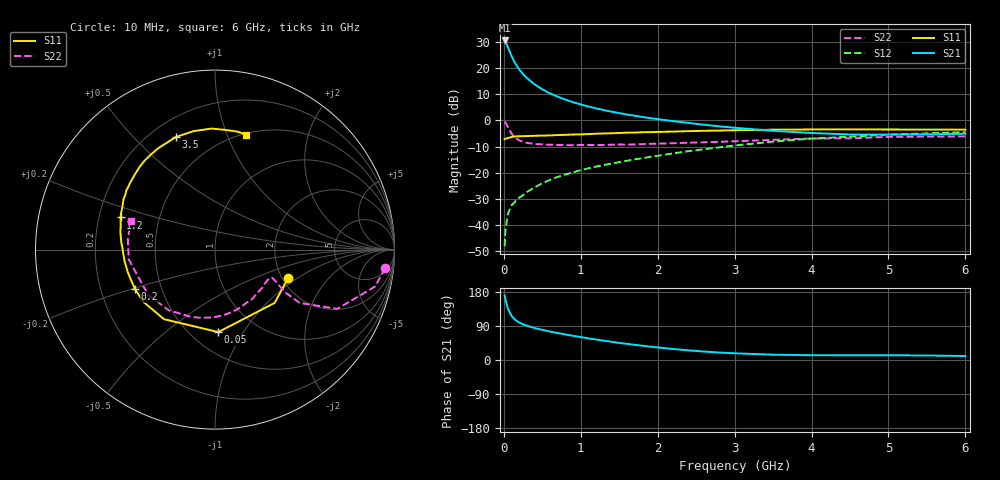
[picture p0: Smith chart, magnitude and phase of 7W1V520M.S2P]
! Infineon Technologies  Discrete & RF Semiconductors
! BFS17W
! Si NPN RF Bipolar Junction Transistor in SOT323
! VCE = 1.5 V  IC = 20 mA
! Common Emitter S-Parameters:  August  1999
# GHz  S  MA  R  50
!  f  S11  S21  S12  S22
! GHz  MAG  ANG  MAG  ANG  MAG  ANG  MAG  ANG
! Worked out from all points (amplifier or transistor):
!   36 points, 10 MHz to 6 GHz, reference 50 ohm
!   highest |S21| = 30.6 dB at 10 MHz (marker M1)
!   |S21| within 3 dB of that: start of sweep to 58.85 MHz
!   unconditionally stable (mu >= 1): 219.1 MHz to end of sweep
!   at 250 MHz: K = 1.08, MAG = 21.5 dB, |S12| = -28.6 dB
!   at 1.4 GHz: K = 1.28, MAG = 6.7 dB, |S12| = -16.5 dB
!   at 6 GHz: K = 1.11, MAG = -2.3 dB, |S12| = -4.5 dB
!   S11 on the Smith chart (normalised r, x): 10 MHz: 2.14, -0.85; 50 MHz: 0.67, -0.78; 200 MHz: 0.35, -0.20; 1.2 GHz: 0.29, +0.15; 3.5 GHz: 0.30, +0.67; 6 GHz: 0.51, +1.18
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0.01  0.4366 -21.6  34.02 170.0  0.0039 83.4  0.9538 -6.2
0.02  0.4456 -41.8  32.74 159.9  0.0075 74.6  0.9152 -13.0
0.05  0.4599 -87.7  25.94 136.8  0.0159 61.6  0.7565 -25.9
0.1  0.4806 -126.2  17.05 116.3  0.0235 54.6  0.5571 -32.2
0.15  0.4944 -144.1  12.26 105.5  0.0282 55.6  0.4611 -31.4
0.2  0.4971 -153.9  9.496 99.0  0.0332 58.4  0.4148 -29.5
0.25  0.498 -160.8  7.702 94.2  0.0371 60.0  0.3861 -27.9
0.3  0.5018 -165.5  6.476 90.5  0.0425 61.5  0.3724 -27.1
0.4  0.5078 -172.6  4.908 84.3  0.0523 63.7  0.3533 -26.3
0.5  0.5118 -177.6  3.947 79.5  0.0624 66.1  0.3469 -26.7
0.6  0.5159 178.9  3.293 75.1  0.0727 67.0  0.342 -27.9
0.7  0.524 175.4  2.845 71.1  0.0827 67.7  0.3388 -30.0
0.9  0.5368 169.3  2.232 63.8  0.1013 68.1  0.3358 -34.9
1.1  0.5481 163.6  1.846 57.0  0.1211 68.0  0.3377 -41.0
1.2  0.5561 161.2  1.701 54.0  0.1305 67.7  0.3373 -44.3
1.6  0.5828 150.8  1.297 42.6  0.1689 67.4  0.3439 -58.2
2.2  0.6115 137.1  0.97 29.0  0.2334 65.6  0.3662 -80.5
2.8  0.6396 123.7  0.77 19.7  0.3049 61.2  0.3889 -102.8
3.5  0.6643 109.1  0.632 14.0  0.3931 53.7  0.4251 -127.4
4.5  0.6747 91.7  0.538 12.4  0.4891 40.4  0.4543 -161.0
5.5  0.669 79.4  0.54 11.9  0.5658 28.6  0.4895 172.8
6  0.6647 74.7  0.555 10.5  0.5963 23.1  0.4951 161.3
